FUNCTION FC 119 : VOID
TITLE =DATA FOR OP_37 FOR VISUALIZE STATUS MONITORING.
AUTHOR : Esposito
FAMILY : EGAL_srl
NAME : MONITOR
VERSION : 0.1

BEGIN
NETWORK
TITLE =BIT, SIGNAL LEVEL ZERO
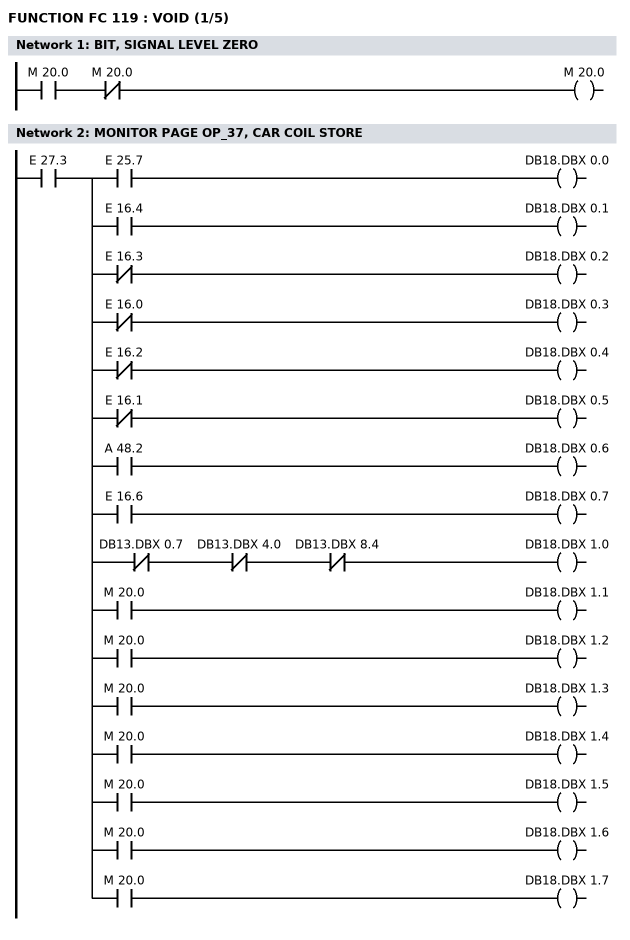
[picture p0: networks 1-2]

      U     M     20.0;
      UN    M     20.0;
      =     M     20.0;
NETWORK
TITLE =MONITOR PAGE OP_37, CAR COIL STORE

      U     E     27.3;
      =     L      0.0;
      U     L      0.0;
      U     E     25.7;
      =     DB18.DBX    0.0;
      U     L      0.0;
      U     E     16.4;
      =     DB18.DBX    0.1;
      U     L      0.0;
      UN    E     16.3;
      =     DB18.DBX    0.2;
      U     L      0.0;
      UN    E     16.0;
      =     DB18.DBX    0.3;
      U     L      0.0;
      UN    E     16.2;
      =     DB18.DBX    0.4;
      U     L      0.0;
      UN    E     16.1;
      =     DB18.DBX    0.5;
      U     L      0.0;
      U     A     48.2;
      =     DB18.DBX    0.6;
      U     L      0.0;
      U     E     16.6;
      =     DB18.DBX    0.7;
      U     L      0.0;
      UN    DB13.DBX    0.7;
      UN    DB13.DBX    4.0;
      UN    DB13.DBX    8.4;
      =     DB18.DBX    1.0;
      U     L      0.0;
      U     M     20.0;
      =     DB18.DBX    1.1;
      U     L      0.0;
      U     M     20.0;
      =     DB18.DBX    1.2;
      U     L      0.0;
      U     M     20.0;
      =     DB18.DBX    1.3;
      U     L      0.0;
      U     M     20.0;
      =     DB18.DBX    1.4;
      U     L      0.0;
      U     M     20.0;
      =     DB18.DBX    1.5;
      U     L      0.0;
      U     M     20.0;
      =     DB18.DBX    1.6;
      U     L      0.0;
      U     M     20.0;
      =     DB18.DBX    1.7;
NETWORK
TITLE =MONITOR PAGE OP_37, ASPO (REEL)
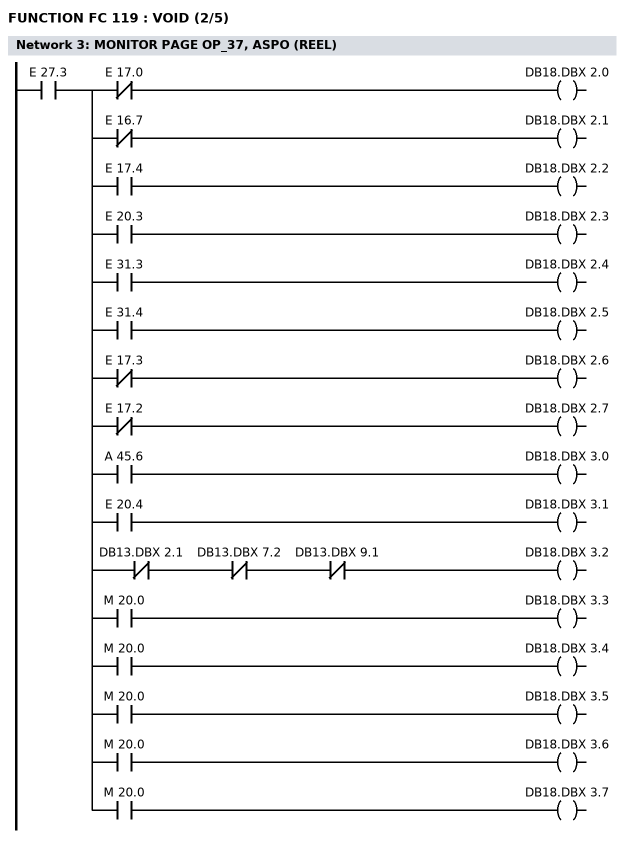
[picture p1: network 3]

      U     E     27.3;
      =     L      0.0;
      U     L      0.0;
      UN    E     17.0;
      =     DB18.DBX    2.0;
      U     L      0.0;
      UN    E     16.7;
      =     DB18.DBX    2.1;
      U     L      0.0;
      U     E     17.4;
      =     DB18.DBX    2.2;
      U     L      0.0;
      U     E     20.3;
      =     DB18.DBX    2.3;
      U     L      0.0;
      U     E     31.3;
      =     DB18.DBX    2.4;
      U     L      0.0;
      U     E     31.4;
      =     DB18.DBX    2.5;
      U     L      0.0;
      UN    E     17.3;
      =     DB18.DBX    2.6;
      U     L      0.0;
      UN    E     17.2;
      =     DB18.DBX    2.7;
      U     L      0.0;
      U     A     45.6;
      =     DB18.DBX    3.0;
      U     L      0.0;
      U     E     20.4;
      =     DB18.DBX    3.1;
      U     L      0.0;
      UN    DB13.DBX    2.1;
      UN    DB13.DBX    7.2;
      UN    DB13.DBX    9.1;
      =     DB18.DBX    3.2;
      U     L      0.0;
      U     M     20.0;
      =     DB18.DBX    3.3;
      U     L      0.0;
      U     M     20.0;
      =     DB18.DBX    3.4;
      U     L      0.0;
      U     M     20.0;
      =     DB18.DBX    3.5;
      U     L      0.0;
      U     M     20.0;
      =     DB18.DBX    3.6;
      U     L      0.0;
      U     M     20.0;
      =     DB18.DBX    3.7;
NETWORK
TITLE =MONITOR PAGE OP_37 STRAIGHTENER
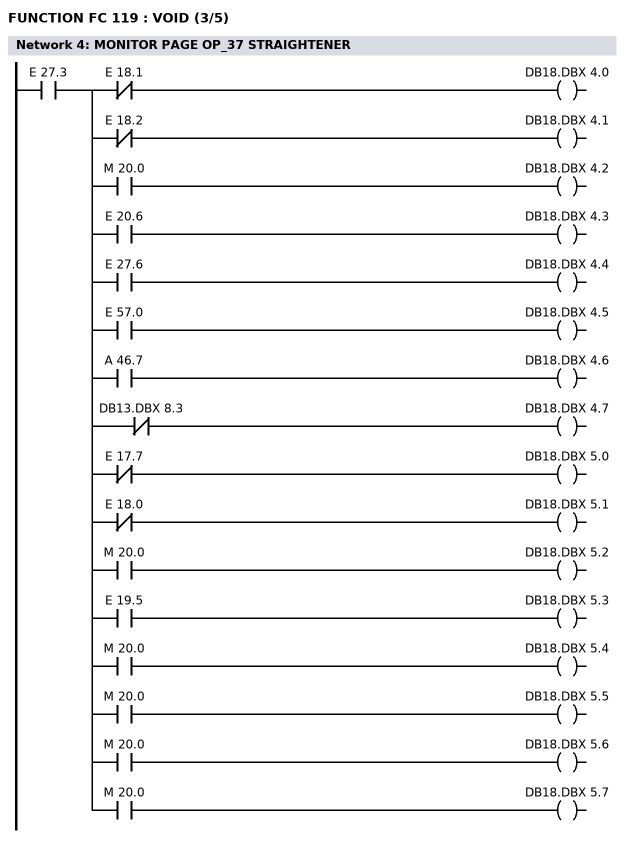
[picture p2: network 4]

      U     E     27.3;
      =     L      0.0;
      U     L      0.0;
      UN    E     18.1;
      =     DB18.DBX    4.0;
      U     L      0.0;
      UN    E     18.2;
      =     DB18.DBX    4.1;
      U     L      0.0;
      U     M     20.0;
      =     DB18.DBX    4.2;
      U     L      0.0;
      U     E     20.6;
      =     DB18.DBX    4.3;
      U     L      0.0;
      U     E     27.6;
      =     DB18.DBX    4.4;
      U     L      0.0;
      U     E     57.0;
      =     DB18.DBX    4.5;
      U     L      0.0;
      U     A     46.7;
      =     DB18.DBX    4.6;
      U     L      0.0;
      UN    DB13.DBX    8.3;
      =     DB18.DBX    4.7;
      U     L      0.0;
      UN    E     17.7;
      =     DB18.DBX    5.0;
      U     L      0.0;
      UN    E     18.0;
      =     DB18.DBX    5.1;
      U     L      0.0;
      U     M     20.0;
      =     DB18.DBX    5.2;
      U     L      0.0;
      U     E     19.5;
      =     DB18.DBX    5.3;
      U     L      0.0;
      U     M     20.0;
      =     DB18.DBX    5.4;
      U     L      0.0;
      U     M     20.0;
      =     DB18.DBX    5.5;
      U     L      0.0;
      U     M     20.0;
      =     DB18.DBX    5.6;
      U     L      0.0;
      U     M     20.0;
      =     DB18.DBX    5.7;
NETWORK
TITLE =MONITOR PAGE OP_37, ANSA
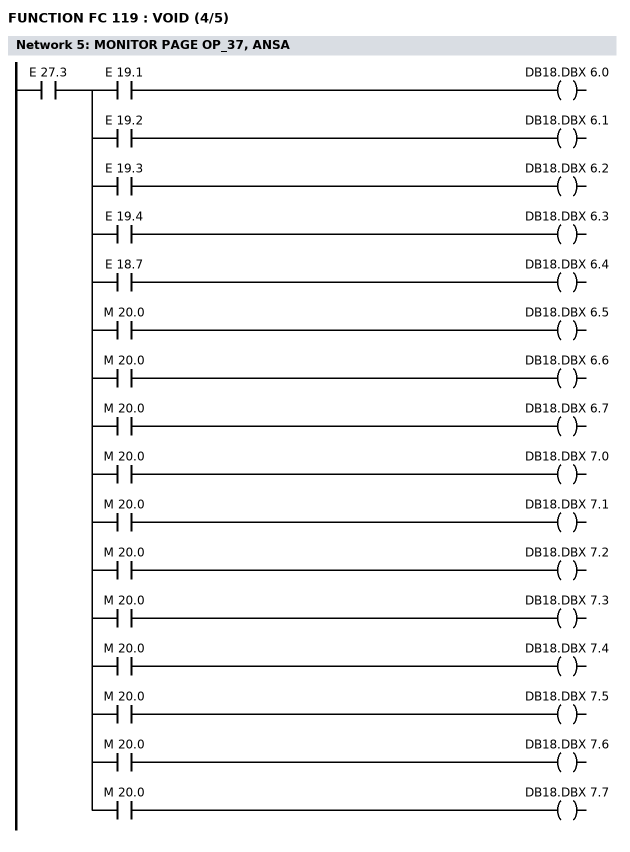
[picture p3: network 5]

      U     E     27.3;
      =     L      0.0;
      U     L      0.0;
      U     E     19.1;
      =     DB18.DBX    6.0;
      U     L      0.0;
      U     E     19.2;
      =     DB18.DBX    6.1;
      U     L      0.0;
      U     E     19.3;
      =     DB18.DBX    6.2;
      U     L      0.0;
      U     E     19.4;
      =     DB18.DBX    6.3;
      U     L      0.0;
      U     E     18.7;
      =     DB18.DBX    6.4;
      U     L      0.0;
      U     M     20.0;
      =     DB18.DBX    6.5;
      U     L      0.0;
      U     M     20.0;
      =     DB18.DBX    6.6;
      U     L      0.0;
      U     M     20.0;
      =     DB18.DBX    6.7;
      U     L      0.0;
      U     M     20.0;
      =     DB18.DBX    7.0;
      U     L      0.0;
      U     M     20.0;
      =     DB18.DBX    7.1;
      U     L      0.0;
      U     M     20.0;
      =     DB18.DBX    7.2;
      U     L      0.0;
      U     M     20.0;
      =     DB18.DBX    7.3;
      U     L      0.0;
      U     M     20.0;
      =     DB18.DBX    7.4;
      U     L      0.0;
      U     M     20.0;
      =     DB18.DBX    7.5;
      U     L      0.0;
      U     M     20.0;
      =     DB18.DBX    7.6;
      U     L      0.0;
      U     M     20.0;
      =     DB18.DBX    7.7;
NETWORK
TITLE =MONITOR PAGE OP_37, FEEDER
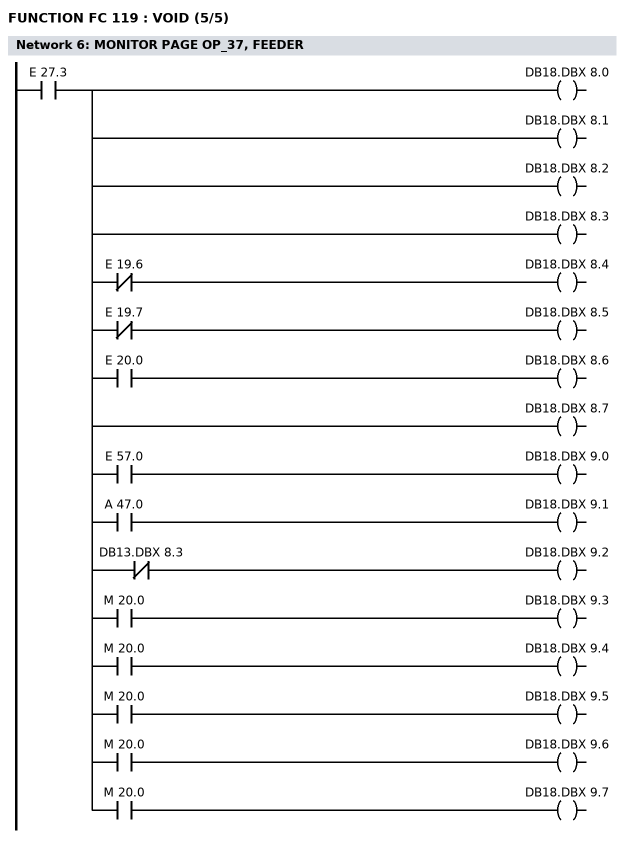
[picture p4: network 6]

      U     E     27.3;
      =     L      0.0;
      U     L      0.0;
      BLD   102;
      =     DB18.DBX    8.0;
      U     L      0.0;
      BLD   102;
      =     DB18.DBX    8.1;
      U     L      0.0;
      BLD   102;
      =     DB18.DBX    8.2;
      U     L      0.0;
      BLD   102;
      =     DB18.DBX    8.3;
      U     L      0.0;
      UN    E     19.6;
      =     DB18.DBX    8.4;
      U     L      0.0;
      UN    E     19.7;
      =     DB18.DBX    8.5;
      U     L      0.0;
      U     E     20.0;
      =     DB18.DBX    8.6;
      U     L      0.0;
      BLD   102;
      =     DB18.DBX    8.7;
      U     L      0.0;
      U     E     57.0;
      =     DB18.DBX    9.0;
      U     L      0.0;
      U     A     47.0;
      =     DB18.DBX    9.1;
      U     L      0.0;
      UN    DB13.DBX    8.3;
      =     DB18.DBX    9.2;
      U     L      0.0;
      U     M     20.0;
      =     DB18.DBX    9.3;
      U     L      0.0;
      U     M     20.0;
      =     DB18.DBX    9.4;
      U     L      0.0;
      U     M     20.0;
      =     DB18.DBX    9.5;
      U     L      0.0;
      U     M     20.0;
      =     DB18.DBX    9.6;
      U     L      0.0;
      U     M     20.0;
      =     DB18.DBX    9.7;
END_FUNCTION

